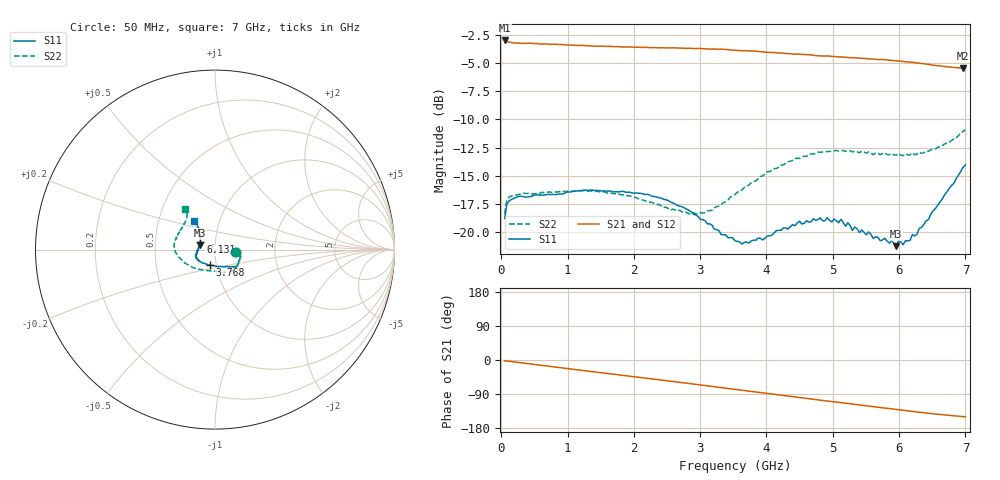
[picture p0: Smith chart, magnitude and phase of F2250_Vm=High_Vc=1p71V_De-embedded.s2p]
! Integrated Device Technology
! Corporate Headquarters
! 6024 Silver Creek Valley Road
! San Jose, CA 95138  USA
! Phone:  1-408-284-8200
! Toll Free:  1-800-223-1366
! Webpage:  http://www.idt.com/
! Timing and RF Division
! 515 Groton Road, Suite 102
! Westford, MA 01886-6024
! Device:  F2250
! Description: Voltage Variable RF Attenuator
! Frequency:  50.0 -  6000.00 MHz
! Package:  3x3 mm Thin QFN Plastic Package: 16 pin
! Ports:  2 RF, 3 DC
!  Pin  1  = GND
!  Pin  2  = NC
!  Pin  3  = RF1  = Port 1
!  Pin  4  = NC
!  Pin  5  = GND
!  Pin  6  = GND
!  Pin  7  = GND
!  Pin  8  = GND
!  Pin  9  = NC
!  Pin 10  = RF2  = Port 2
!  Pin 11  = NC
!  Pin 12  = GND
!  Pin 13  = GND
!  Pin 14  = VCNTRL
!  Pin 15  = VDD
!  Pin 16  = VMODE
! Vcntrl:  1.710 Volts
! Vmode:  +3.300 Volts
! Vdd:  +3.30  Volts
! Current:  1.326 mA
! Data:  The device was measured on a the F2250 evaluation board which has
!  individual transmission lines to the RF pins.  Data was collected
!  using a calibrated network analyzer.  The evaluation board was
!  de-embedded using a TRL calibration technique.
!  The reference plane is the edge of the package pin.
! Misc:  SN 10
!  Action Tracker AT0258
! Date Measured:  2014-11-26
! Date:  2015-10-15  MJV
! Note:
!  Integrated Device Technology supplies this data as a sample of measured
!  data at the package pin for this product.  Your particular data for this
!  product may vary.
!  Data was taken at 25 degrees C.
!  Integrated Device Technology reserves the right to change this data at anytime.
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# GHz S dB R 50
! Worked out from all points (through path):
!   201 points, 50 MHz to 7 GHz, reference 50 ohm
!   highest |S21| = -2.99 dB at 50 MHz (marker M1); lowest = -5.5 dB at 6.965 GHz (marker M2)
!   group delay of S21, straight-line fit = 60.2 ps
!   lowest |S11| = -21.2 dB at 5.957 GHz (marker M3), VSWR 1.19, Z = 42.3 + j2.08 ohm
!   |S11| at or under -10 dB: start of sweep to end of sweep
!   |S22| runs from -18.4 to -10.9 dB; largest |S21 - S12| = 0.0029
!   S11 on the Smith chart (normalised r, x): 50 MHz: 1.26, -0.03; 3.768 GHz: 0.93, -0.16; 6.131 GHz: 0.85, +0.07; 7 GHz: 0.76, +0.25
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0.05  -18.81 -5.3  -2.99 -2.2  -2.99 -2.1  -18.38 -6.4
0.08475  -17.48 -4.3  -3.11 -2.7  -3.11 -2.7  -17.12 -5.4
0.2585  -16.83 -8.9  -3.22 -6.4  -3.23 -6.4  -16.67 -11.9
1.2315  -16.29 -32.9  -3.43 -27.7  -3.43 -27.7  -16.32 -46.2
2.37825  -16.93 -42.0  -3.65 -52.1  -3.65 -52.1  -17.54 -72.2
2.969  -18.61 -53.6  -3.69 -65.1  -3.71 -65.1  -18.41 -99.3
3.525  -20.77 -86.6  -3.85 -77.6  -3.84 -77.6  -16.66 -133.4
3.76825  -20.78 -107.3  -3.93 -83.0  -3.92 -83.1  -15.63 -145.7
4.4285  -19.43 -142.5  -4.21 -97.5  -4.19 -97.6  -13.46 -170.5
4.7065  -18.81 -153.3  -4.29 -103.6  -4.30 -103.6  -13.08 -177.4
5.1235  -18.86 -163.9  -4.45 -112.7  -4.45 -112.7  -12.76 172.3
5.29725  -19.85 -167.9  -4.52 -116.3  -4.50 -116.4  -12.89 168.7
5.332  -19.55 -170.3  -4.53 -117.1  -4.52 -117.2  -12.81 167.7
5.85325  -20.98 170.1  -4.75 -128.2  -4.74 -128.3  -13.13 153.7
5.888  -20.75 169.9  -4.75 -129.0  -4.74 -129.1  -13.01 153.8
5.9575  -21.25 163.6  -4.79 -130.4  -4.79 -130.5  -13.18 151.0
5.99225  -20.77 162.1  -4.81 -131.3  -4.79 -131.4  -13.01 150.6
6.06175  -21.12 157.8  -4.84 -132.6  -4.85 -132.7  -13.22 147.9
6.13125  -20.79 153.3  -4.90 -134.1  -4.87 -134.2  -13.16 145.9
6.444  -18.89 135.6  -5.11 -140.6  -5.09 -140.7  -12.82 135.7
6.96525  -14.25 126.0  -5.47 -149.5  -5.47 -149.6  -11.07 127.4
7  -14.04 125.7  -5.46 -150.0  -5.47 -150.1  -10.93 126.5
